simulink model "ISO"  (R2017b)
settings: Solver=FixedStepDiscrete  StartTime=0.0  StopTime=10.0  FixedStep=0.01  RelTol=1e-3  EnableMultiTasking=on
undefined symbols (not defined in the file): ASWTYPE_FALSE, ASWTYPE_TRUE, CcISO_CTCOnlineDelayTime_ms, CcISO_FirLvlDebTime_ms, CcISO_FirLvlResChrg_kohm, CcISO_FirLvlResNotChrg_kohm, CcISO_InitDiagDebMaxTi_ms, CcISO_InitDiagDebTi_ms, CcISO_IsoDefaultValue_kohm, CcISO_IsoFastDectectInsVal_kohm, CcISO_IsoFastDetectCnf_MS, CcISO_IsoFastDetectVal_kohm, CcISO_IsoMeasDelayTime_ms, CcISO_ISONegVoltDebTime_ms, CcISO_ISONegVoltFliterDiff_V, CcISO_ISOPackVoltMax_V, CcISO_ISOPackVoltMin_V, CcISO_ISOResCnfFltCnt_NUMB, CcISO_ISOResCnfFltVal_kohm, CcISO_ISOResCnfWarnCnt_NUMB, CcISO_ISOResCnfWarnVal_kohm, CcISO_ISOResNvmMin_kohm, CcISO_ISOResValueinit_kohm, CcISO_IsoResVldVal_NUMB, CcISO_ISOSlopeDelayTime_ms, CcISO_ISOSlopeFilterVal_NUMB, CcISO_NegStMeasFiltTi_ms, CcISO_NegVoltHighRat_pct, CcISO_NegVoltLowRat_pct, CcISO_NorLvlResChrg_kohm, CcISO_NorLvlResNotChrg_kohm, CcISO_PosStMeasFiltTi_ms, CcISO_ResSelfCheckDebTime_ms, CcISO_SedLvlDebTime_ms, CcISO_SedLvlResChrg_kohm, CcISO_SedLvlResNotChrg_kohm, Enum_CTCCtrCtlConnMode, Enum_CTCCtrCtlState, Enum_ISOHVIsoFltLevel, Enum_ISOHVIsoMeasState, Enum_LDPCC2St, Enum_MSMBMUState, ISO_CONST0_NUMB, ISO_CONST1000_NUMB, ISO_CONST1_NUMB, ISO_RESRB1_OHM, ISO_RESRB2_OHM, ISO_RESRS1_OHM, ISO_RESRS2_OHM, ISO_RUNTIME_MS
libraries: AIWAYS_Powertrain_BMS_lib x49
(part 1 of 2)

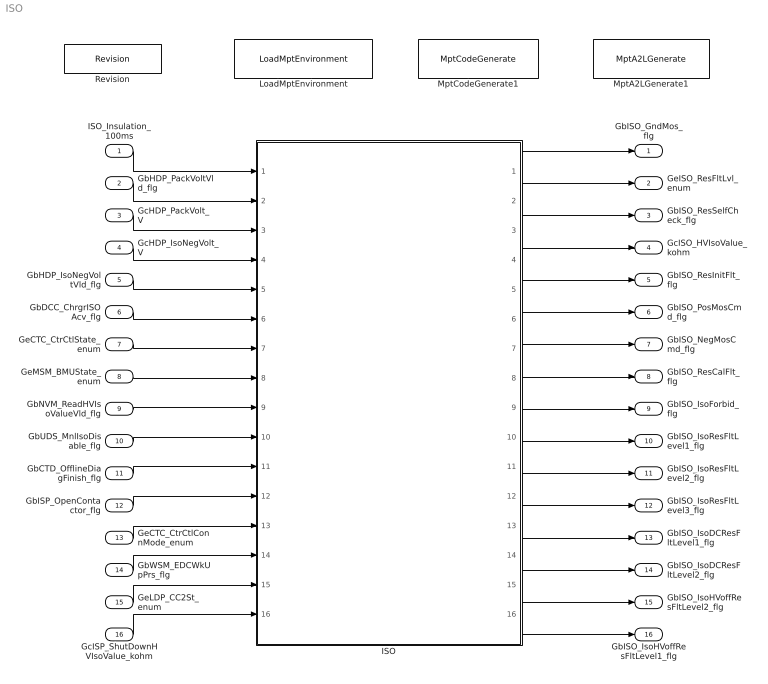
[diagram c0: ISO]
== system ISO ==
  ISO_Insulation_100ms : Inport
  GbHDP_PackVoltVld_flg : Inport  Port=2
  GcHDP_PackVolt_V : Inport  Port=3
  GcHDP_IsoNegVolt_V : Inport  Port=4
  GbHDP_IsoNegVoltVld_flg : Inport  Port=5
  GbDCC_ChrgrISOAcv_flg : Inport  Port=6
  GeCTC_CtrCtlState_enum : Inport  Port=7
  GeMSM_BMUState_enum : Inport  Port=8
  GbNVM_ReadHVIsoValueVld_flg : Inport  Port=9
  GbUDS_MnlIsoDisable_flg : Inport  Port=10
  GbCTD_OfflineDiagFinish_flg : Inport  Port=11
  GbISP_OpenContactor_flg : Inport  Port=12
  GeCTC_CtrCtlConnMode_enum : Inport  Port=13
  GbWSM_EDCWkUpPrs_flg : Inport  Port=14
  GeLDP_CC2St_enum : Inport  Port=15
  GcISP_ShutDownHVIsoValue_kohm : Inport  Port=16
  ISO : Subsystem
  LoadMptEnvironment : AIWAYS_Powertrain_BMS_lib/Config/LoadMptEnvironment  ProjectName=Comm  SuppierID=NewPlatformUAES
  MptA2LGenerate1 : AIWAYS_Powertrain_BMS_lib/Config/MptA2LGenerate  SystemSampleTime=-1
  MptCodeGenerate1 : AIWAYS_Powertrain_BMS_lib/Config/MptCodeGenerate  SystemSampleTime=-1
  Revision : AIWAYS_Powertrain_BMS_lib/Config/Revision  curVersion='M114C112R114'  newVersion='M114C112R114'
  GbISO_GndMos_flg : Outport
  GeISO_ResFltLvl_enum : Outport  Port=2
  GbISO_ResSelfCheck_flg : Outport  Port=3
  GcISO_HVIsoValue_kohm : Outport  Port=4
  GbISO_ResInitFlt_flg : Outport  Port=5
  GbISO_PosMosCmd_flg : Outport  Port=6
  GbISO_NegMosCmd_flg : Outport  Port=7
  GbISO_ResCalFlt_flg : Outport  Port=8
  GbISO_IsoForbid_flg : Outport  Port=9
  GbISO_IsoResFltLevel1_flg : Outport  Port=10
  GbISO_IsoResFltLevel2_flg : Outport  Port=11
  GbISO_IsoResFltLevel3_flg : Outport  Port=12
  GbISO_IsoDCResFltLevel1_flg : Outport  Port=13
  GbISO_IsoDCResFltLevel2_flg : Outport  Port=14
  GbISO_IsoHVoffResFltLevel2_flg : Outport  Port=15
  GbISO_IsoHVoffResFltLevel1_flg : Outport  Port=16
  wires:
  ISO_Insulation_100ms/1 -> ISO/1(ISO_Insulation_100ms)
  GbHDP_PackVoltVld_flg/1 -> ISO/2(GbHDP_PackVoltVld_flg)
  GcHDP_PackVolt_V/1 -> ISO/3(GcHDP_PackVolt_V)
  GcHDP_IsoNegVolt_V/1 -> ISO/4(GcHDP_IsoNegVolt_V)
  GbHDP_IsoNegVoltVld_flg/1 -> ISO/5(GbHDP_IsoNegVoltVld_flg)
  GbDCC_ChrgrISOAcv_flg/1 -> ISO/6(GbDCC_ChrgrISOAcv_flg)
  GeCTC_CtrCtlState_enum/1 -> ISO/7(GeCTC_CtrCtlState_enum)
  GeMSM_BMUState_enum/1 -> ISO/8(GeMSM_BMUState_enum)
  GbNVM_ReadHVIsoValueVld_flg/1 -> ISO/9(GbNVM_ReadHVIsoValueVld_flg)
  GbUDS_MnlIsoDisable_flg/1 -> ISO/10(GbUDS_MnlIsoDisable_flg)
  GbCTD_OfflineDiagFinish_flg/1 -> ISO/11(GbCTD_OfflineDiagFinish_flg)
  GbISP_OpenContactor_flg/1 -> ISO/12(GbISP_OpenContactor_flg)
  GeCTC_CtrCtlConnMode_enum/1 -> ISO/13(GeCTC_CtrCtlConnMode_enum)
  ISO/1(GbISO_GndMos_flg) -> GbISO_GndMos_flg/1
  ISO/2(GeISO_ResFltLvl_enum) -> GeISO_ResFltLvl_enum/1
  ISO/3(GbISO_ResSelfCheck_flg) -> GbISO_ResSelfCheck_flg/1
  ISO/4(GcISO_HVIsoValue_kohm) -> GcISO_HVIsoValue_kohm/1
  ISO/5(GbISO_ResInitFlt_flg) -> GbISO_ResInitFlt_flg/1
  ISO/6(GbISO_PosMosCmd_flg) -> GbISO_PosMosCmd_flg/1
  ISO/7(GbISO_NegMosCmd_flg) -> GbISO_NegMosCmd_flg/1
  ISO/8(GbISO_ResCalFlt_flg) -> GbISO_ResCalFlt_flg/1
  GbWSM_EDCWkUpPrs_flg/1 -> ISO/14(GbWSM_EDCWkUpPrs_flg)
  ISO/9(GbISO_IsoForbid_flg) -> GbISO_IsoForbid_flg/1
  ISO/10(GbISO_IsoResFltLevel1_flg) -> GbISO_IsoResFltLevel1_flg/1
  ISO/11(GbISO_IsoResFltLevel2_flg) -> GbISO_IsoResFltLevel2_flg/1
  ISO/12(GbISO_IsoResFltLevel3_flg) -> GbISO_IsoResFltLevel3_flg/1
  GeLDP_CC2St_enum/1 -> ISO/15(GeLDP_CC2St_enum)
  ISO/13(GbISO_IsoDCResFltLevel1_flg) -> GbISO_IsoDCResFltLevel1_flg/1
  ISO/14(GbISO_IsoDCResFltLevel2_flg) -> GbISO_IsoDCResFltLevel2_flg/1
  ISO/15(GbISO_IsoHVoffResFltLevel2_flg) -> GbISO_IsoHVoffResFltLevel2_flg/1
  ISO/16(GbISO_IsoHVoffResFltLevel1_flg) -> GbISO_IsoHVoffResFltLevel1_flg/1
  GcISP_ShutDownHVIsoValue_kohm/1 -> ISO/16(GcISP_ShutDownHVIsoValue_kohm)

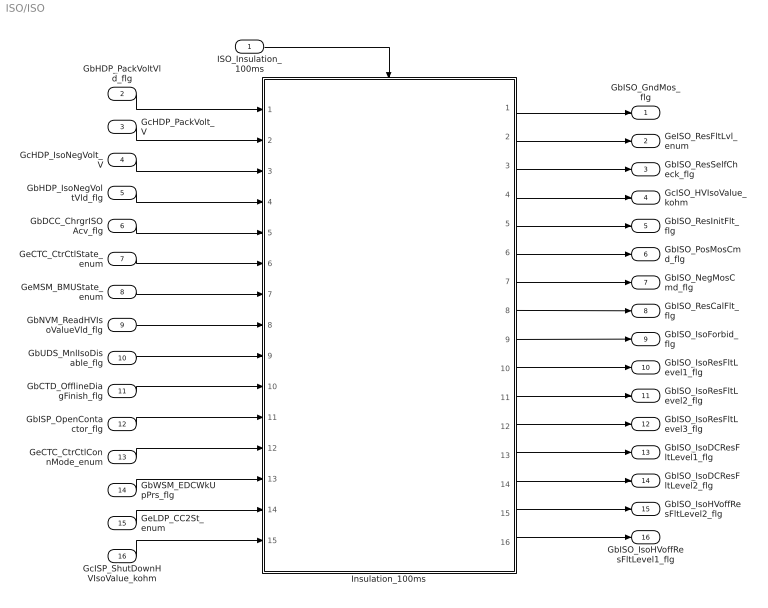
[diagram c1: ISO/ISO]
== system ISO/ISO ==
  ISO_Insulation_100ms : Inport
  GbHDP_PackVoltVld_flg : Inport  Port=2
  GcHDP_PackVolt_V : Inport  Port=3
  GcHDP_IsoNegVolt_V : Inport  Port=4
  GbHDP_IsoNegVoltVld_flg : Inport  Port=5
  GbDCC_ChrgrISOAcv_flg : Inport  Port=6
  GeCTC_CtrCtlState_enum : Inport  Port=7
  GeMSM_BMUState_enum : Inport  Port=8
  GbNVM_ReadHVIsoValueVld_flg : Inport  Port=9
  GbUDS_MnlIsoDisable_flg : Inport  Port=10
  GbCTD_OfflineDiagFinish_flg : Inport  Port=11
  GbISP_OpenContactor_flg : Inport  Port=12
  GeCTC_CtrCtlConnMode_enum : Inport  Port=13
  GbWSM_EDCWkUpPrs_flg : Inport  Port=14
  GeLDP_CC2St_enum : Inport  Port=15
  GcISP_ShutDownHVIsoValue_kohm : Inport  Port=16
  Insulation_100ms : Subsystem
  GbISO_GndMos_flg : Outport
  GeISO_ResFltLvl_enum : Outport  Port=2
  GbISO_ResSelfCheck_flg : Outport  Port=3
  GcISO_HVIsoValue_kohm : Outport  Port=4
  GbISO_ResInitFlt_flg : Outport  Port=5
  GbISO_PosMosCmd_flg : Outport  Port=6
  GbISO_NegMosCmd_flg : Outport  Port=7
  GbISO_ResCalFlt_flg : Outport  Port=8
  GbISO_IsoForbid_flg : Outport  Port=9
  GbISO_IsoResFltLevel1_flg : Outport  Port=10
  GbISO_IsoResFltLevel2_flg : Outport  Port=11
  GbISO_IsoResFltLevel3_flg : Outport  Port=12
  GbISO_IsoDCResFltLevel1_flg : Outport  Port=13
  GbISO_IsoDCResFltLevel2_flg : Outport  Port=14
  GbISO_IsoHVoffResFltLevel2_flg : Outport  Port=15
  GbISO_IsoHVoffResFltLevel1_flg : Outport  Port=16
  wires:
  ISO_Insulation_100ms/1 -> Insulation_100ms/Trigger
  Insulation_100ms/1(GbISO_GndMos_flg) -> GbISO_GndMos_flg/1
  Insulation_100ms/2(GeISO_ResFltLvl_enum) -> GeISO_ResFltLvl_enum/1
  Insulation_100ms/3(GbISO_ResSelfCheck_flg) -> GbISO_ResSelfCheck_flg/1
  Insulation_100ms/4(GcISO_HVIsoValue_kohm) -> GcISO_HVIsoValue_kohm/1
  Insulation_100ms/5(GbISO_ResInitFlt_flg) -> GbISO_ResInitFlt_flg/1
  Insulation_100ms/6(GbISO_PosMosCmd_flg) -> GbISO_PosMosCmd_flg/1
  Insulation_100ms/7(GbISO_NegMosCmd_flg) -> GbISO_NegMosCmd_flg/1
  Insulation_100ms/8(GbISO_ResCalFlt_flg) -> GbISO_ResCalFlt_flg/1
  GbHDP_PackVoltVld_flg/1 -> Insulation_100ms/1(GbHDP_PackVoltVld_flg)
  GcHDP_PackVolt_V/1 -> Insulation_100ms/2(GcHDP_PackVolt_V)
  GcHDP_IsoNegVolt_V/1 -> Insulation_100ms/3(GcHDP_IsoNegVolt_V)
  GbHDP_IsoNegVoltVld_flg/1 -> Insulation_100ms/4(GbHDP_IsoNegVoltVld_flg)
  GbDCC_ChrgrISOAcv_flg/1 -> Insulation_100ms/5(GbDCC_ChrgrISOAcv_flg)
  GeCTC_CtrCtlState_enum/1 -> Insulation_100ms/6(GeCTC_CtrCtlState_enum)
  GeMSM_BMUState_enum/1 -> Insulation_100ms/7(GeMSM_BMUState_enum)
  GbNVM_ReadHVIsoValueVld_flg/1 -> Insulation_100ms/8(GbNVM_ReadHVIsoValueVld_flg)
  GbUDS_MnlIsoDisable_flg/1 -> Insulation_100ms/9(GbUDS_MnlIsoDisable_flg)
  GbCTD_OfflineDiagFinish_flg/1 -> Insulation_100ms/10(GbCTD_OfflineDiagFinish_flg)
  GbISP_OpenContactor_flg/1 -> Insulation_100ms/11(GbISP_OpenContactor_flg)
  GeCTC_CtrCtlConnMode_enum/1 -> Insulation_100ms/12(GeCTC_CtrCtlConnMode_enum)
  GbWSM_EDCWkUpPrs_flg/1 -> Insulation_100ms/13(GbWSM_EDCWkUpPrs_flg)
  Insulation_100ms/9(GbISO_IsoForbid_flg) -> GbISO_IsoForbid_flg/1
  Insulation_100ms/10(GbISO_IsoResFltLevel1_flg) -> GbISO_IsoResFltLevel1_flg/1
  Insulation_100ms/11(GbISO_IsoResFltLevel2_flg) -> GbISO_IsoResFltLevel2_flg/1
  Insulation_100ms/12(GbISO_IsoResFltLevel3_flg) -> GbISO_IsoResFltLevel3_flg/1
  GeLDP_CC2St_enum/1 -> Insulation_100ms/14(GeLDP_CC2St_enum)
  Insulation_100ms/13(GbISO_IsoDCResFltLevel1_flg) -> GbISO_IsoDCResFltLevel1_flg/1
  Insulation_100ms/14(GbISO_IsoDCResFltLevel2_flg) -> GbISO_IsoDCResFltLevel2_flg/1
  Insulation_100ms/15(GbISO_IsoHVoffResFltLevel2_flg) -> GbISO_IsoHVoffResFltLevel2_flg/1
  Insulation_100ms/16(GbISO_IsoHVoffResFltLevel1_flg) -> GbISO_IsoHVoffResFltLevel1_flg/1
  GcISP_ShutDownHVIsoValue_kohm/1 -> Insulation_100ms/15(GcISP_ShutDownHVIsoValue_kohm)

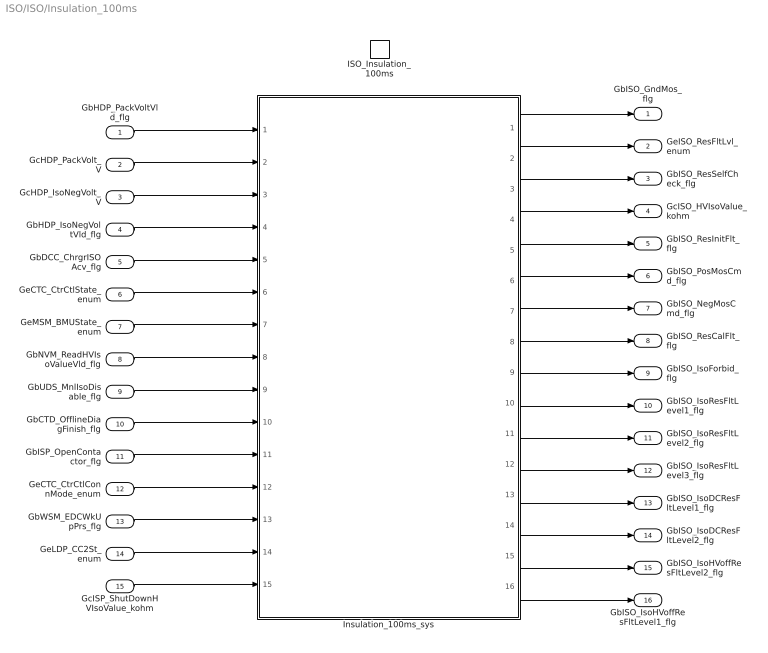
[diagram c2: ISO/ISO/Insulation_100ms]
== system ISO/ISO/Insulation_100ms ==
  GbHDP_PackVoltVld_flg : Inport
  GcHDP_PackVolt_V : Inport  Port=2
  GcHDP_IsoNegVolt_V : Inport  Port=3
  GbHDP_IsoNegVoltVld_flg : Inport  Port=4
  GbDCC_ChrgrISOAcv_flg : Inport  Port=5
  GeCTC_CtrCtlState_enum : Inport  Port=6
  GeMSM_BMUState_enum : Inport  Port=7
  GbNVM_ReadHVIsoValueVld_flg : Inport  Port=8
  GbUDS_MnlIsoDisable_flg : Inport  Port=9
  GbCTD_OfflineDiagFinish_flg : Inport  Port=10
  GbISP_OpenContactor_flg : Inport  Port=11
  GeCTC_CtrCtlConnMode_enum : Inport  Port=12
  GbWSM_EDCWkUpPrs_flg : Inport  Port=13
  GeLDP_CC2St_enum : Inport  Port=14
  GcISP_ShutDownHVIsoValue_kohm : Inport  Port=15
  ISO_Insulation_100ms : TriggerPort  TriggerType=function-call  VariantControl=(inherit)
  Insulation_100ms_sys : Subsystem
  GbISO_GndMos_flg : Outport
  GeISO_ResFltLvl_enum : Outport  Port=2
  GbISO_ResSelfCheck_flg : Outport  Port=3
  GcISO_HVIsoValue_kohm : Outport  Port=4
  GbISO_ResInitFlt_flg : Outport  Port=5
  GbISO_PosMosCmd_flg : Outport  Port=6
  GbISO_NegMosCmd_flg : Outport  Port=7
  GbISO_ResCalFlt_flg : Outport  Port=8
  GbISO_IsoForbid_flg : Outport  Port=9
  GbISO_IsoResFltLevel1_flg : Outport  Port=10
  GbISO_IsoResFltLevel2_flg : Outport  Port=11
  GbISO_IsoResFltLevel3_flg : Outport  Port=12
  GbISO_IsoDCResFltLevel1_flg : Outport  Port=13
  GbISO_IsoDCResFltLevel2_flg : Outport  Port=14
  GbISO_IsoHVoffResFltLevel2_flg : Outport  Port=15
  GbISO_IsoHVoffResFltLevel1_flg : Outport  Port=16
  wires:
  Insulation_100ms_sys/1(GbISO_GndMos_flg) -> GbISO_GndMos_flg/1
  Insulation_100ms_sys/2(GeISO_ResFltLvl_enum) -> GeISO_ResFltLvl_enum/1
  Insulation_100ms_sys/3(GbISO_ResSelfCheck_flg) -> GbISO_ResSelfCheck_flg/1
  Insulation_100ms_sys/4(GcISO_HVIsoValue_kohm) -> GcISO_HVIsoValue_kohm/1
  Insulation_100ms_sys/5(GbISO_ResInitFlt_flg) -> GbISO_ResInitFlt_flg/1
  Insulation_100ms_sys/6(GbISO_PosMosCmd_flg) -> GbISO_PosMosCmd_flg/1
  Insulation_100ms_sys/7(GbISO_NegMosCmd_flg) -> GbISO_NegMosCmd_flg/1
  Insulation_100ms_sys/8(GbISO_ResCalFlt_flg) -> GbISO_ResCalFlt_flg/1
  GbHDP_PackVoltVld_flg/1 -> Insulation_100ms_sys/1(GbHDP_PackVoltVld_flg)
  GcHDP_PackVolt_V/1 -> Insulation_100ms_sys/2(GcHDP_PackVolt_V)
  GcHDP_IsoNegVolt_V/1 -> Insulation_100ms_sys/3(GcHDP_IsoNegVolt_V)
  GbHDP_IsoNegVoltVld_flg/1 -> Insulation_100ms_sys/4(GbHDP_IsoNegVoltVld_flg)
  GbDCC_ChrgrISOAcv_flg/1 -> Insulation_100ms_sys/5(GbDCC_ChrgrISOAcv_flg)
  GeCTC_CtrCtlState_enum/1 -> Insulation_100ms_sys/6(GeCTC_CtrCtlState_enum)
  GeMSM_BMUState_enum/1 -> Insulation_100ms_sys/7(GeMSM_BMUState_enum)
  GbNVM_ReadHVIsoValueVld_flg/1 -> Insulation_100ms_sys/8(GbNVM_ReadHVIsoValueVld_flg)
  GbUDS_MnlIsoDisable_flg/1 -> Insulation_100ms_sys/9(GbUDS_MnlIsoDisable_flg)
  GbCTD_OfflineDiagFinish_flg/1 -> Insulation_100ms_sys/10(GbCTD_OfflineDiagFinish_flg)
  GbISP_OpenContactor_flg/1 -> Insulation_100ms_sys/11(GbISP_OpenContactor_flg)
  GeCTC_CtrCtlConnMode_enum/1 -> Insulation_100ms_sys/12(GeCTC_CtrCtlConnMode_enum)
  GbWSM_EDCWkUpPrs_flg/1 -> Insulation_100ms_sys/13(GbWSM_EDCWkUpPrs_flg)
  Insulation_100ms_sys/9(GbISO_IsoForbid_flg) -> GbISO_IsoForbid_flg/1
  Insulation_100ms_sys/10(GbISO_IsoResFltLevel1_flg) -> GbISO_IsoResFltLevel1_flg/1
  Insulation_100ms_sys/11(GbISO_IsoResFltLevel2_flg) -> GbISO_IsoResFltLevel2_flg/1
  Insulation_100ms_sys/12(GbISO_IsoResFltLevel3_flg) -> GbISO_IsoResFltLevel3_flg/1
  GeLDP_CC2St_enum/1 -> Insulation_100ms_sys/14(GeLDP_CC2St_enum)
  Insulation_100ms_sys/13(GbISO_IsoDCResFltLevel1_flg) -> GbISO_IsoDCResFltLevel1_flg/1
  Insulation_100ms_sys/14(GbISO_IsoDCResFltLevel2_flg) -> GbISO_IsoDCResFltLevel2_flg/1
  Insulation_100ms_sys/15(GbISO_IsoHVoffResFltLevel2_flg) -> GbISO_IsoHVoffResFltLevel2_flg/1
  Insulation_100ms_sys/16(GbISO_IsoHVoffResFltLevel1_flg) -> GbISO_IsoHVoffResFltLevel1_flg/1
  GcISP_ShutDownHVIsoValue_kohm/1 -> Insulation_100ms_sys/15(GcISP_ShutDownHVIsoValue_kohm)

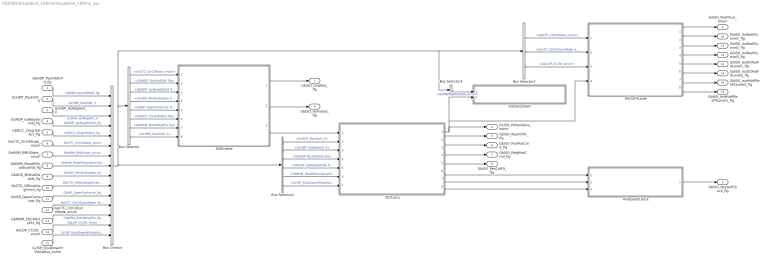
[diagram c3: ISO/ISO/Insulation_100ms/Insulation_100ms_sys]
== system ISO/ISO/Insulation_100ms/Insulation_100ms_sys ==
  GbHDP_PackVoltVld_flg : Inport
  GcHDP_PackVolt_V : Inport  Port=2
  GcHDP_IsoNegVolt_V : Inport  Port=3
  GbHDP_IsoNegVoltVld_flg : Inport  Port=4
  GbDCC_ChrgrISOAcv_flg : Inport  Port=5
  GeCTC_CtrCtlState_enum : Inport  Port=6
  GeMSM_BMUState_enum : Inport  Port=7
  GbNVM_ReadHVIsoValueVld_flg : Inport  Port=8
  GbUDS_MnlIsoDisable_flg : Inport  Port=9
  GbCTD_OfflineDiagFinish_flg : Inport  Port=10
  GbISP_OpenContactor_flg : Inport  Port=11
  GeCTC_CtrCtlConnMode_enum : Inport  Port=12
  GbWSM_EDCWkUpPrs_flg : Inport  Port=13
  GeLDP_CC2St_enum : Inport  Port=14
  GcISP_ShutDownHVIsoValue_kohm : Inport  Port=15
  Bus Creator : BusCreator  Inputs=15
  Bus Selector : BusSelector  OutputSignals=GeCTC_CtrCtlState_enum,GbHDP_PackVoltVld_flg,GbHDP_IsoNegVoltVld_flg,GbUDS_MnlIsoDisable_flg,GbISP_OpenContactor_flg,GbDCC_ChrgrISOAcv_flg,GbWSM_EDCWkUpPrs_flg,GcHDP_PackVolt_V
  Bus Selector1 : BusSelector  OutputSignals=GcHDP_PackVolt_V,GcHDP_IsoNegVolt_V,GbHDP_PackVoltVld_flg,GbHDP_IsoNegVoltVld_flg,GbNVM_ReadHVIsoValueVld_flg,GcISP_ShutDownHVIsoValue_kohm
  Bus Selector2 : BusSelector  OutputSignals=GeCTC_CtrCtlState_enum,GeCTC_CtrCtlConnMode_enum,GeLDP_CC2St_enum
  Bus Selector3 : BusSelector  OutputSignals=GeMSM_BMUState_enum
  DataStoreISO : Subsystem
  HVIsoFltLevel : Subsystem
  HVIsoSelfCheck : Subsystem
  ISOCalcu : Subsystem
  ISOEnable : Subsystem
  GbISO_GndMos_flg : Outport
  GeISO_ResFltLvl_enum : Outport  Port=2
  GbISO_ResSelfCheck_flg : Outport  Port=3
  GcISO_HVIsoValue_kohm : Outport  Port=4
  GbISO_ResInitFlt_flg : Outport  Port=5
  GbISO_PosMosCmd_flg : Outport  Port=6
  GbISO_NegMosCmd_flg : Outport  Port=7
  GbISO_ResCalFlt_flg : Outport  Port=8
  GbISO_IsoForbid_flg : Outport  Port=9
  GbISO_IsoResFltLevel1_flg : Outport  Port=10
  GbISO_IsoResFltLevel2_flg : Outport  Port=11
  GbISO_IsoResFltLevel3_flg : Outport  Port=12
  GbISO_IsoDCResFltLevel1_flg : Outport  Port=13
  GbISO_IsoDCResFltLevel2_flg : Outport  Port=14
  GbISO_IsoHVoffResFltLevel2_flg : Outport  Port=15
  GbISO_IsoHVoffResFltLevel1_flg : Outport  Port=16
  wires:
  GbHDP_PackVoltVld_flg/1 -> Bus Creator/1  "GbHDP_PackVoltVld_flg"
  GcHDP_PackVolt_V/1 -> Bus Creator/2  "GcHDP_PackVolt_V"
  GcHDP_IsoNegVolt_V/1 -> Bus Creator/3  "GcHDP_IsoNegVolt_V"
  GbHDP_IsoNegVoltVld_flg/1 -> Bus Creator/4  "GbHDP_IsoNegVoltVld_flg"
  GbDCC_ChrgrISOAcv_flg/1 -> Bus Creator/5  "GbDCC_ChrgrISOAcv_flg"
  GeCTC_CtrCtlState_enum/1 -> Bus Creator/6  "GeCTC_CtrCtlState_enum"
  GeMSM_BMUState_enum/1 -> Bus Creator/7  "GeMSM_BMUState_enum"
  GbNVM_ReadHVIsoValueVld_flg/1 -> Bus Creator/8  "GbNVM_ReadHVIsoValueVld_flg"
  GbUDS_MnlIsoDisable_flg/1 -> Bus Creator/9  "GbUDS_MnlIsoDisable_flg"
  GbCTD_OfflineDiagFinish_flg/1 -> Bus Creator/10  "GbCTD_OfflineDiagFinish_flg"
  Bus Selector/1 -> ISOEnable/1(GeCTC_CtrCtlState_enum)  "<GeCTC_CtrCtlState_enum>"
  Bus Selector/2 -> ISOEnable/2(GbHDP_PackVoltVld_flg)  "<GbHDP_PackVoltVld_flg>"
  Bus Selector/3 -> ISOEnable/3(GbHDP_IsoNegVoltVld_flg)  "<GbHDP_IsoNegVoltVld_flg>"
  Bus Selector/4 -> ISOEnable/4(GbUDS_MnlIsoDisable_flg)  "<GbUDS_MnlIsoDisable_flg>"
  Bus Selector/5 -> ISOEnable/5(GbISP_OpenContactor_flg)  "<GbISP_OpenContactor_flg>"
  Bus Selector/6 -> ISOEnable/6(GbDCC_ChrgrISOAcv_flg)  "<GbDCC_ChrgrISOAcv_flg>"
  ISOEnable/3(LbISO_IsoForbid_flg) -> ISOCalcu/1(LbISO_IsoForbid_flg)
  Bus Selector1/1 -> ISOCalcu/2(GcHDP_PackVolt_V)  "<GcHDP_PackVolt_V>"
  Bus Selector1/2 -> ISOCalcu/3(GcHDP_IsoNegVolt_V)  "<GcHDP_IsoNegVolt_V>"
  Bus Selector1/3 -> ISOCalcu/4(GbHDP_PackVoltVld_flg)  "<GbHDP_PackVoltVld_flg>"
  Bus Selector1/4 -> ISOCalcu/5(GbHDP_IsoNegVoltVld_flg)  "<GbHDP_IsoNegVoltVld_flg>"
  ISOEnable/1(GbISO_GndMos_flg) -> GbISO_GndMos_flg/1
  Bus Selector1/5 -> ISOCalcu/6(GbNVM_ReadHVIsoValueVld_flg)  "<GbNVM_ReadHVIsoValueVld_flg>"
  ISOCalcu/1(GcISO_HVIsoValue_kohm) -> DataStoreISO/2(GcISO_HVIsoValue_kohm), HVIsoFltLevel/4(GcISO_HVIsoValue_kohm), GcISO_HVIsoValue_kohm/1
  GeCTC_CtrCtlConnMode_enum/1 -> Bus Creator/12  "GeCTC_CtrCtlConnMode_enum"
  Bus Selector2/1 -> HVIsoFltLevel/1(GeCTC_CtrCtlState_enum)  "<GeCTC_CtrCtlState_enum>"
  Bus Selector2/2 -> HVIsoFltLevel/2(GeCTC_CtrCtlConnMode_enum)  "<GeCTC_CtrCtlConnMode_enum>"
  Bus Creator/1 -> Bus Selector3/1, Bus Selector2/1, Bus Selector/1, Bus Selector1/1
  Bus Selector3/1 -> DataStoreISO/1(GeMSM_BMUState_enum)  "<GeMSM_BMUState_enum>"
  HVIsoFltLevel/1(GeISO_ResFltLvl_enum) -> GeISO_ResFltLvl_enum/1
  HVIsoSelfCheck/1(GbISO_ResSelfCheck_flg) -> GbISO_ResSelfCheck_flg/1
  ISOCalcu/2(GbISO_ResInitFlt_flg) -> GbISO_ResInitFlt_flg/1
  ISOCalcu/3(GbISO_PosMosCmd_flg) -> GbISO_PosMosCmd_flg/1
  ISOCalcu/4(GbISO_NegMosCmd_flg) -> GbISO_NegMosCmd_flg/1
  ISOCalcu/5(GbISO_ResCalFlt_flg) -> GbISO_ResCalFlt_flg/1
  GbWSM_EDCWkUpPrs_flg/1 -> Bus Creator/13  "GbWSM_EDCWkUpPrs_flg"
  Bus Selector/7 -> ISOEnable/7(GbWSM_EDCWkUpPrs_flg)  "<GbWSM_EDCWkUpPrs_flg>"
  ISOEnable/2(GbISO_IsoForbid_flg) -> GbISO_IsoForbid_flg/1
  HVIsoFltLevel/2(GbISO_IsoResFltLevel1_flg) -> GbISO_IsoResFltLevel1_flg/1
  HVIsoFltLevel/3(GbISO_IsoResFltLevel2_flg) -> GbISO_IsoResFltLevel2_flg/1
  HVIsoFltLevel/4(GbISO_IsoResFltLevel3_flg) -> GbISO_IsoResFltLevel3_flg/1
  Bus Selector/8 -> ISOEnable/8(" GcHDP_PackVolt_V")  "<GcHDP_PackVolt_V>"
  GbISP_OpenContactor_flg/1 -> Bus Creator/11  "GbISP_OpenContactor_flg"
  GeLDP_CC2St_enum/1 -> Bus Creator/14  "GeLDP_CC2St_enum"
  Bus Selector2/3 -> HVIsoFltLevel/3(GeLDP_CC2St_enum)  "<GeLDP_CC2St_enum>"
  HVIsoFltLevel/5(GbISO_IsoDCResFltLevel1_flg) -> GbISO_IsoDCResFltLevel1_flg/1
  HVIsoFltLevel/6(GbISO_IsoDCResFltLevel2_flg) -> GbISO_IsoDCResFltLevel2_flg/1
  HVIsoFltLevel/7(GbISO_IsoHVoffResFltLevel2_flg) -> GbISO_IsoHVoffResFltLevel2_flg/1
  HVIsoFltLevel/8(GbISO_IsoHVoffResFltLevel1_flg) -> GbISO_IsoHVoffResFltLevel1_flg/1
  ISOCalcu/6(LbISO_InitNegVoltCheck_flg) -> HVIsoSelfCheck/1(LbISO_InitNegVoltCheck_flg)
  ISOCalcu/7(LbISO_IsoFastDetectEna_flg) -> HVIsoSelfCheck/2(LbISO_IsoFastDetectEna_flg)
  GcISP_ShutDownHVIsoValue_kohm/1 -> Bus Creator/15  "GcISP_ShutDownHVIsoValue_kohm"
  Bus Selector1/6 -> ISOCalcu/7(GcISP_ShutDownHVIsoValue_kohm)  "<GcISP_ShutDownHVIsoValue_kohm>"
  ISOCalcu/8(LcISO_HVIsoValue_kohm) -> HVIsoSelfCheck/3(LcISO_HVIsoValue_kohm)

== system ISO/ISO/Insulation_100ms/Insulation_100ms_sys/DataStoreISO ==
  GeMSM_BMUState_enum : Inport
  GcISO_HVIsoValue_kohm : Inport  Port=2
  Constant3 : Constant  Value=Enum_MSMBMUState.Enum_MSMBMUState_Shutdown
  Data Type Conversion1 : DataTypeConversion
  DataStoreISO_Work : Subsystem
  Relational Operator3 : RelationalOperator  Operator===  OutDataTypeStr=boolean
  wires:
  GcISO_HVIsoValue_kohm/1 -> DataStoreISO_Work/1(GcISO_HVIsoValue_kohm)
  GeMSM_BMUState_enum/1 -> Data Type Conversion1/1
  Relational Operator3/1 -> DataStoreISO_Work/Enable  "LbISO_DataStoreEN_flg"
  Constant3/1 -> Relational Operator3/2
  Data Type Conversion1/1 -> Relational Operator3/1

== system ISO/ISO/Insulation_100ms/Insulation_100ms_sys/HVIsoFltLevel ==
  GeCTC_CtrCtlState_enum : Inport
  GeCTC_CtrCtlConnMode_enum : Inport  Port=2
  GeLDP_CC2St_enum : Inport  Port=3
  GcISO_HVIsoValue_kohm : Inport  Port=4
  ISOFlt : Subsystem
  IsoLevelResThrld : Subsystem
  GeISO_ResFltLvl_enum : Outport
  GbISO_IsoResFltLevel1_flg : Outport  Port=2
  GbISO_IsoResFltLevel2_flg : Outport  Port=3
  GbISO_IsoResFltLevel3_flg : Outport  Port=4
  GbISO_IsoDCResFltLevel1_flg : Outport  Port=5
  GbISO_IsoDCResFltLevel2_flg : Outport  Port=6
  GbISO_IsoHVoffResFltLevel2_flg : Outport  Port=7
  GbISO_IsoHVoffResFltLevel1_flg : Outport  Port=8
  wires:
  GcISO_HVIsoValue_kohm/1 -> ISOFlt/1(GcISO_HVIsoValue_kohm)
  GeCTC_CtrCtlState_enum/1 -> IsoLevelResThrld/1(GeCTC_CtrCtlState_enum), ISOFlt/3(GeCTC_CtrCtlState_enum)
  IsoLevelResThrld/1(LcISO_IsoSecondLevelResThrld_kohm) -> ISOFlt/4(LcISO_IsoSecondLevelResThrld_kohm)
  IsoLevelResThrld/2(LcISO_IsoFirstLevelResThrld_kohm) -> ISOFlt/5(LcISO_IsoFirstLevelResThrld_kohm)
  IsoLevelResThrld/3(LcISO_IsoNormalLevelResThrld_kohm) -> ISOFlt/6(LcISO_IsoNormalLevelResThrld_kohm)
  GeCTC_CtrCtlConnMode_enum/1 -> IsoLevelResThrld/2(GeCTC_CtrCtlConnMode_enum)
  ISOFlt/1(GeISO_ResFltLvl_enum) -> GeISO_ResFltLvl_enum/1
  ISOFlt/2(GbISO_IsoResFltLevel1_flg) -> GbISO_IsoResFltLevel1_flg/1
  ISOFlt/3(GbISO_IsoResFltLevel2_flg) -> GbISO_IsoResFltLevel2_flg/1
  ISOFlt/4(GbISO_IsoResFltLevel3_flg) -> GbISO_IsoResFltLevel3_flg/1
  GeLDP_CC2St_enum/1 -> ISOFlt/2(GeLDP_CC2St_enum)
  ISOFlt/5(GbISO_IsoDCResFltLevel1_flg) -> GbISO_IsoDCResFltLevel1_flg/1
  ISOFlt/6(GbISO_IsoDCResFltLevel2_flg) -> GbISO_IsoDCResFltLevel2_flg/1
  ISOFlt/7(GbISO_IsoHVoffResFltLevel2_flg) -> GbISO_IsoHVoffResFltLevel2_flg/1
  ISOFlt/8(GbISO_IsoHVoffResFltLevel1_flg) -> GbISO_IsoHVoffResFltLevel1_flg/1

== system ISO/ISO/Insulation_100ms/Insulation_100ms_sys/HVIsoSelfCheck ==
  LbISO_InitNegVoltCheck_flg : Inport
  LbISO_IsoFastDetectEna_flg : Inport  Port=2
  LcISO_HVIsoValue_kohm : Inport  Port=3
  BMSDebounceStartZero : AIWAYS_Powertrain_BMS_lib/Debounce & Delay/BMSDebounceStartZero
  Comparison : RelationalOperator  Operator=>  OutDataTypeStr=boolean
  Comparison1 : RelationalOperator  Operator===  OutDataTypeStr=boolean
  Comparison2 : RelationalOperator  Operator===  OutDataTypeStr=boolean
  Comparison4 : RelationalOperator  Operator===  OutDataTypeStr=boolean
  Constant1 : Constant  Value=ASWTYPE_TRUE
  Constant2 : Constant  Value=ASWTYPE_TRUE
  Constant3 : Constant  Value=ASWTYPE_FALSE
  Constant4 : Constant  Value=CcISO_ResSelfCheckDebTime_ms
  Constant5 : Constant  Value=ISO_RUNTIME_MS
  Constant6 : Constant  Value=ISO_RUNTIME_MS
  Constant7 : Constant  Value=CcISO_ResSelfCheckDebTime_ms
  Constant8 : Constant  Value=CcISO_ISOResCnfFltVal_kohm
  ISO_GbISO_ResSelfCheck_flg : AIWAYS_Powertrain_BMS_lib/Signals/OverWrite  OverWrite_Value=CbISO_ResSelfCheckOvr_flg  OverWrite_flag=CbISO_ResSelfCheckOvrSwt_flg
  Logical : Logic  OutDataTypeStr=boolean
  Logical1 : Logic  Operator=OR  Inputs=3  OutDataTypeStr=boolean
  GbISO_ResSelfCheck_flg : Outport
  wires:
  Logical1/1 -> BMSDebounceStartZero/1
  ISO_GbISO_ResSelfCheck_flg/1 -> GbISO_ResSelfCheck_flg/1  "GbISO_ResSelfCheck_flg"
  Constant1/1 -> Comparison4/2
  Constant2/1 -> Comparison1/2
  LbISO_InitNegVoltCheck_flg/1 -> Comparison1/1
  Comparison4/1 -> Logical/2
  Comparison1/1 -> Logical/1
  Logical/1 -> Logical1/1
  Comparison2/1 -> Logical1/2
  Constant3/1 -> Comparison2/2
  LbISO_IsoFastDetectEna_flg/1 -> Comparison4/1, Comparison2/1
  BMSDebounceStartZero/1 -> ISO_GbISO_ResSelfCheck_flg/1
  Constant6/1 -> BMSDebounceStartZero/3
  Constant4/1 -> BMSDebounceStartZero/2
  Constant5/1 -> BMSDebounceStartZero/5
  Constant7/1 -> BMSDebounceStartZero/4
  LcISO_HVIsoValue_kohm/1 -> Comparison/1
  Comparison/1 -> Logical1/3
  Constant8/1 -> Comparison/2

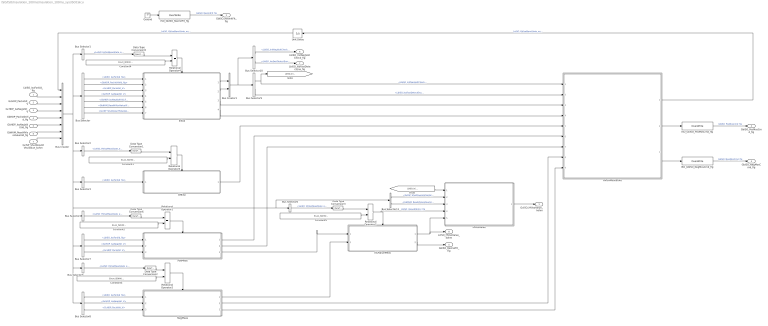
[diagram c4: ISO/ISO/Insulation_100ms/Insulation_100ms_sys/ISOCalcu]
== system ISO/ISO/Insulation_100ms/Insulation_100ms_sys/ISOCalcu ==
  LbISO_IsoForbid_flg : Inport
  GcHDP_PackVolt_V : Inport  Port=2
  GcHDP_IsoNegVolt_V : Inport  Port=3
  GbHDP_PackVoltVld_flg : Inport  Port=4
  GbHDP_IsoNegVoltVld_flg : Inport  Port=5
  GbNVM_ReadHVIsoValueVld_flg : Inport  Port=6
  GcISP_ShutDownHVIsoValue_kohm : Inport  Port=7
  Bus Creator : BusCreator  Inputs=8
  Bus Creator1 : BusCreator  Inputs=2
  Bus Selector : BusSelector  OutputSignals=LbISO_IsoForbid_flg,GbHDP_PackVoltVld_flg,GcHDP_PackVolt_V,GcHDP_IsoNegVolt_V,GbHDP_IsoNegVoltVld_flg,GbNVM_ReadHVIsoValueVld_flg,GcISP_ShutDownHVIsoValue_kohm
  Bus Selector{1..2,4..6} (5 alike) : BusSelector  OutputSignals=LeISO_HVIsoMeasState_enum
  Bus Selector10 : BusSelector  OutputSignals=LbISO_InitNegVoltCheck_flg,LbISO_IsoFastDetectEna_flg
  Bus Selector11 : BusSelector  OutputSignals=GcISP_ShutDownHVIsoValue_kohm,GbNVM_ReadHVIsoValueVld_flg
  Bus Selector3 : BusSelector  OutputSignals=LbISO_IsoForbid_flg
  Bus Selector7 : BusSelector  OutputSignals=LbISO_IsoForbid_flg,GcHDP_IsoNegVolt_V,GcHDP_PackVolt_V
  Bus Selector8 : BusSelector  OutputSignals=LbISO_IsoForbid_flg,GcHDP_IsoNegVolt_V,GcHDP_PackVolt_V
  Bus Selector9 : BusSelector  OutputSignals=LbISO_InitNegVoltCheck_flg,LbISO_IsoFastDetectEna_flg
  Constant1 : Constant  Value=Enum_ISOHVIsoMeasState.Enum_ISOHVIsoMeasState_Offline
  Constant2 : Constant  Value=Enum_ISOHVIsoMeasState.Enum_ISOHVIsoMeasState_PosMeas
  Constant3 : Constant  Value=Enum_ISOHVIsoMeasState.Enum_ISOHVIsoMeasState_NegMeas
  Constant4 : Constant  Value=Enum_ISOHVIsoMeasState.Enum_ISOHVIsoMeasState_Initial
  Constant5 : Constant  Value=Enum_ISOHVIsoMeasState.Enum_ISOHVIsoMeasState_VauleCalcu
  Data Type Conversion{1..3,5..6} (5 alike) : DataTypeConversion
  Ground : Ground
  HVIsoMeasState : Stateflow chart  TreatAsAtomicUnit=on
  HVIsoValue : Subsystem
  ISOValueMeas : Subsystem  TreatAsAtomicUnit=on
  ISO_GbISO_NegMosCmd_flg : AIWAYS_Powertrain_BMS_lib/Signals/OverWrite  OverWrite_Value=CbISO_NegMosCmdOvr_flg  OverWrite_flag=CbISO_NegMosCmdOvrSwt_flg
  ISO_GbISO_PosMosCmd_flg : AIWAYS_Powertrain_BMS_lib/Signals/OverWrite  OverWrite_Value=CbISO_PosMosCmdOvr_flg  OverWrite_flag=CbISO_PosMosCmdOvrSwt_flg
  ISO_GbISO_ResInitFlt_flg : AIWAYS_Powertrain_BMS_lib/Signals/OverWrite  OverWrite_Value=CbISO_ResInitFltOvr_flg  OverWrite_flag=CbISO_ResInitFltOvrSwt_flg
  Initial : Subsystem  TreatAsAtomicUnit=on
  NegMeas : Subsystem  TreatAsAtomicUnit=on
  Offline : Subsystem  TreatAsAtomicUnit=on
  PosMeas : Subsystem  TreatAsAtomicUnit=on
  Relational Operator{1..5} (5 alike) : RelationalOperator  Operator===  OutDataTypeStr=boolean
  Unit Delay : UnitDelay  SampleTime=-1  StateName=StateName
  GcISO_HVIsoValue_kohm : Outport
  GbISO_ResInitFlt_flg : Outport  Port=2
  GbISO_PosMosCmd_flg : Outport  Port=3
  GbISO_NegMosCmd_flg : Outport  Port=4
  GbISO_ResCalFlt_flg : Outport  Port=5
  LbISO_InitNegVoltCheck_flg : Outport  Port=6
  LbISO_IsoFastDetectEna_flg : Outport  Port=7
  LcISO_HVIsoValue_kohm : Outport  Port=8
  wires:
  Relational Operator1/1 -> PosMeas/Enable
  Relational Operator2/1 -> NegMeas/Enable
  Constant2/1 -> Relational Operator1/2
  Constant3/1 -> Relational Operator2/2
  HVIsoMeasState/2(GbISO_PosMosCmd_flg) -> ISO_GbISO_PosMosCmd_flg/1
  HVIsoMeasState/3(GbISO_NegMosCmd_flg) -> ISO_GbISO_NegMosCmd_flg/1
  ISOValueMeas/1(LcISO_HVIsoValue_kohm) -> LcISO_HVIsoValue_kohm/1, HVIsoValue/5(LcISO_HVIsoValue_kohm)
  HVIsoMeasState/1(LeISO_HVIsoMeasState_enum) -> Unit Delay/1  "LeISO_HVIsoMeasState_enum"
  Data Type Conversion6/1 -> Relational Operator1/1
  Data Type Conversion2/1 -> Relational Operator2/1
  PosMeas/3(LcISO_PosStBeta_numb) -> ISOValueMeas/1(LcISO_PosStBeta_numb)
  NegMeas/1(LcISO_NegStAlpha_numb) -> ISOValueMeas/2(LcISO_NegStAlpha_numb)
  HVIsoValue/1(GcISO_HVIsoValue_kohm) -> GcISO_HVIsoValue_kohm/1
  LbISO_IsoForbid_flg/1 -> Bus Creator/2
  GcHDP_PackVolt_V/1 -> Bus Creator/3
  GcHDP_IsoNegVolt_V/1 -> Bus Creator/4
  GbHDP_PackVoltVld_flg/1 -> Bus Creator/5
  GbHDP_IsoNegVoltVld_flg/1 -> Bus Creator/6
  Unit Delay/1 -> Bus Creator/1  "LeISO_HVIsoMeasState_enum"
  Bus Selector/1 -> Initial/1(LbISO_IsoForbid_flg)  "<LbISO_IsoForbid_flg>"
  Bus Selector/2 -> Initial/2(GbHDP_PackVoltVld_flg)  "<GbHDP_PackVoltVld_flg>"
  Bus Selector/3 -> Initial/3(GcHDP_PackVolt_V)  "<GcHDP_PackVolt_V>"
  Bus Selector/4 -> Initial/4(GcHDP_IsoNegVolt_V)  "<GcHDP_IsoNegVolt_V>"
  Bus Selector/5 -> Initial/5(GbHDP_IsoNegVoltVld_flg)  "<GbHDP_IsoNegVoltVld_flg>"
  Relational Operator4/1 -> Initial/Enable
  Constant4/1 -> Relational Operator4/2
  Data Type Conversion5/1 -> Relational Operator4/1
  Bus Selector1/1 -> Data Type Conversion5/1  "<LeISO_HVIsoMeasState_enum>"
  Bus Selector2/1 -> Data Type Conversion1/1  "<LeISO_HVIsoMeasState_enum>"
  Data Type Conversion1/1 -> Relational Operator5/1
  Constant1/1 -> Relational Operator5/2
  Relational Operator5/1 -> Offline/Enable
  Bus Selector3/1 -> Offline/1(LbISO_IsoForbid_flg)  "<LbISO_IsoForbid_flg>"
  Bus Selector4/1 -> Data Type Conversion6/1  "<LeISO_HVIsoMeasState_enum>"
  Bus Selector5/1 -> Data Type Conversion2/1  "<LeISO_HVIsoMeasState_enum>"
  Bus Selector6/1 -> Data Type Conversion3/1  "<LeISO_HVIsoMeasState_enum>"
  Bus Creator/1 -> Bus Selector1/1, Bus Selector/1, Bus Selector8/1, Bus Selector5/1, Bus Selector7/1, Bus Selector4/1, Bus Selector11/1, Bus Selector6/1, Bus Selector3/1, Bus Selector2/1
  Data Type Conversion3/1 -> Relational Operator3/1
  Constant5/1 -> Relational Operator3/2
  Relational Operator3/1 -> HVIsoValue/4(LbISO_ValueStEntry_flg), ISOValueMeas/Enable  "LbISO_ValueStEntry_flg"
  Initial/3(LbISO_InitiaStMosCmd_flg) -> HVIsoMeasState/3(LbISO_InitiaStMosCmd_flg)
  Initial/4(LbISO_Init2Offline_flg) -> HVIsoMeasState/4(LbISO_Init2Offline_flg)
  Offline/1(LbISO_Offline2PosMeas_flg) -> HVIsoMeasState/5(LbISO_Offline2PosMeas_flg)
  PosMeas/1(LbISO_PosMeas2NegMeas_flg) -> HVIsoMeasState/6(LbISO_PosMeas2NegMeas_flg)
  PosMeas/2(LbISO_PosMeas2Offline_flg) -> HVIsoMeasState/7(LbISO_PosMeas2Offline_flg)
  NegMeas/2(LbISO_NegMeas2VauleCalcu_flg) -> HVIsoMeasState/8(LbISO_NegMeas2VauleCalcu_flg)
  NegMeas/3(LbISO_NegMeas2Offline_flg) -> HVIsoMeasState/9(LbISO_NegMeas2Offline_flg)
  Bus Selector7/1 -> PosMeas/1(LbISO_IsoForbid_flg)  "<LbISO_IsoForbid_flg>"
  Bus Selector7/2 -> PosMeas/2(GcHDP_IsoNegVolt_V)  "<GcHDP_IsoNegVolt_V>"
  Bus Selector7/3 -> PosMeas/3(GcHDP_PackVolt_V)  "<GcHDP_PackVolt_V>"
  Bus Selector8/2 -> NegMeas/2(GcHDP_IsoNegVolt_V)  "<GcHDP_IsoNegVolt_V>"
  Bus Selector8/1 -> NegMeas/1(LbISO_IsoForbid_flg)  "<LbISO_IsoForbid_flg>"
  Bus Selector8/3 -> NegMeas/3(GcHDP_PackVolt_V)  "<GcHDP_PackVolt_V>"
  ISO_GbISO_PosMosCmd_flg/1 -> GbISO_PosMosCmd_flg/1  "GbISO_PosMosCmd_flg"
  ISO_GbISO_NegMosCmd_flg/1 -> GbISO_NegMosCmd_flg/1  "GbISO_NegMosCmd_flg"
  ISOValueMeas/2(GbISO_ResCalFlt_flg) -> GbISO_ResCalFlt_flg/1
  Ground/1 -> ISO_GbISO_ResInitFlt_flg/1
  ISO_GbISO_ResInitFlt_flg/1 -> GbISO_ResInitFlt_flg/1  "GbISO_ResInitFlt_flg"
  GbNVM_ReadHVIsoValueVld_flg/1 -> Bus Creator/7
  Bus Selector/6 -> Initial/6(GbNVM_ReadHVIsoValueVld_flg)  "<GbNVM_ReadHVIsoValueVld_flg>"
  Bus Selector9/2 -> HVIsoMeasState/2(LbISO_IsoFastDetectEna_flg)  "<LbISO_IsoFastDetectEna_flg>"
  Bus Selector9/1 -> [LbISO_InitNegVoltCheck_flg], HVIsoMeasState/1(LbISO_InitNegVoltCheck_flg)  "<LbISO_InitNegVoltCheck_flg>"
  [LbISO_InitNegVoltCheck_flg] -> HVIsoValue/1(LbISO_InitNegVoltCheck_flg)
  Initial/1(LbISO_InitNegVoltCheck_flg) -> Bus Creator1/1
  Initial/2(LbISO_IsoFastDetectEna_flg) -> Bus Creator1/2
  Bus Creator1/1 -> Bus Selector9/1, Bus Selector10/1
  Bus Selector10/1 -> LbISO_InitNegVoltCheck_flg/1  "<LbISO_InitNegVoltCheck_flg>"
  Bus Selector10/2 -> LbISO_IsoFastDetectEna_flg/1  "<LbISO_IsoFastDetectEna_flg>"
  GcISP_ShutDownHVIsoValue_kohm/1 -> Bus Creator/8
  Bus Selector/7 -> Initial/7(GcISP_ShutDownHVIsoValue_kohm)  "<GcISP_ShutDownHVIsoValue_kohm>"
  Bus Selector11/1 -> HVIsoValue/2(GcISP_ShutDownHVIsoValue_kohm)  "<GcISP_ShutDownHVIsoValue_kohm>"
  Bus Selector11/2 -> HVIsoValue/3(GbNVM_ReadHVIsoValueVld_flg)  "<GbNVM_ReadHVIsoValueVld_flg>"

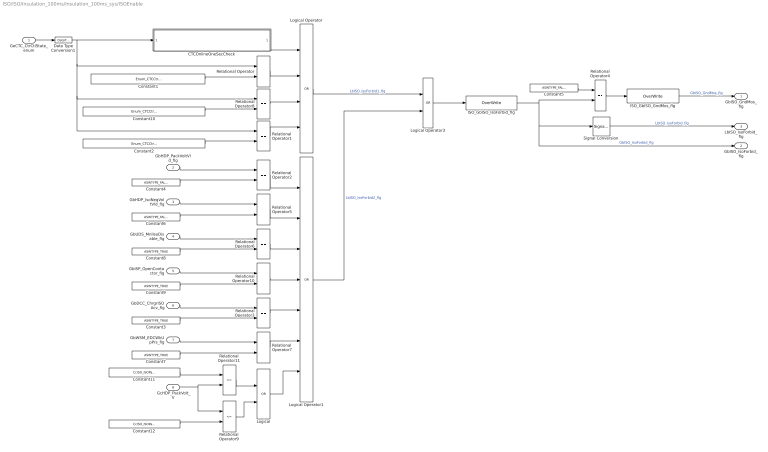
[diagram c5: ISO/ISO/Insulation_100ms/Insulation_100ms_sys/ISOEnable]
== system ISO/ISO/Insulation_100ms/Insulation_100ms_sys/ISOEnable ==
  GeCTC_CtrCtlState_enum : Inport
  GbHDP_PackVoltVld_flg : Inport  Port=2
  GbHDP_IsoNegVoltVld_flg : Inport  Port=3
  GbUDS_MnlIsoDisable_flg : Inport  Port=4
  GbISP_OpenContactor_flg : Inport  Port=5
  GbDCC_ChrgrISOAcv_flg : Inport  Port=6
  GbWSM_EDCWkUpPrs_flg : Inport  Port=7
  " GcHDP_PackVolt_V" : Inport  Port=8
  CTCOnlineOneSecCheck : Subsystem
  Constant1 : Constant  Value=Enum_CTCCtrCtlState.Enum_CTCCtrCtlState_Connect
  Constant10 : Constant  Value=Enum_CTCCtrCtlState.Enum_CTCCtrCtlState_PreShutdown
  Constant11 : Constant  Value=CcISO_ISOPackVoltMax_V
  Constant12 : Constant  Value=CcISO_ISOPackVoltMin_V
  Constant2 : Constant  Value=Enum_CTCCtrCtlState.Enum_CTCCtrCtlState_Shutdown
  Constant{3,7..9} (4 alike) : Constant  Value=ASWTYPE_TRUE
  Constant4 : Constant  Value=ASWTYPE_FALSE
  Constant5 : Constant  Value=ASWTYPE_FALSE
  Constant6 : Constant  Value=ASWTYPE_FALSE
  Data Type Conversion1 : DataTypeConversion
  ISO_GbISO_GndMos_flg : AIWAYS_Powertrain_BMS_lib/Signals/OverWrite  OverWrite_Value=CbISO_GndMosOvr_flg  OverWrite_flag=CbISO_GndMosOvrSwt_flg
  ISO_GbISO_IsoForbid_flg : AIWAYS_Powertrain_BMS_lib/Signals/OverWrite  OverWrite_Value=CbISO_IsoForbidOvr_flg  OverWrite_flag=CbISO_IsoForbidOvrSwt_flg
  Logical : Logic  Operator=OR  OutDataTypeStr=boolean
  Logical Operator : Logic  Operator=OR  Inputs=4  AllPortsSameDT=off  OutDataTypeStr=boolean
  Logical Operator1 : Logic  Operator=OR  Inputs=7  AllPortsSameDT=off  OutDataTypeStr=boolean
  Logical Operator3 : Logic  Operator=OR  AllPortsSameDT=off  OutDataTypeStr=boolean
  Relational Operator{,1..8,10} (10 alike) : RelationalOperator  Operator===  OutDataTypeStr=boolean
  Relational Operator11 : RelationalOperator  Operator=<=  OutDataTypeStr=boolean
  Relational Operator9 : RelationalOperator  Operator=<=  OutDataTypeStr=boolean
  Signal Conversion : SignalConversion  ConversionOutput=Contiguous copy  OverrideOpt=off
  GbISO_GndMos_flg : Outport
  GbISO_IsoForbid_flg : Outport  Port=2
  LbISO_IsoForbid_flg : Outport  Port=3
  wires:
  Constant1/1 -> Relational Operator/2
  Constant2/1 -> Relational Operator1/2
  GbHDP_PackVoltVld_flg/1 -> Relational Operator2/1
  Constant4/1 -> Relational Operator2/2
  GbHDP_IsoNegVoltVld_flg/1 -> Relational Operator5/1
  Constant6/1 -> Relational Operator5/2
  Logical Operator/1 -> Logical Operator3/1  "LbISO_IsoForbid1_flg"
  Logical Operator1/1 -> Logical Operator3/2  "LbISO_IsoForbid2_flg"
  GeCTC_CtrCtlState_enum/1 -> Data Type Conversion1/1
  GbUDS_MnlIsoDisable_flg/1 -> Relational Operator6/1
  Constant8/1 -> Relational Operator6/2
  Data Type Conversion1/1 -> CTCOnlineOneSecCheck/1(GeCTC_CtrCtlState_enum), Relational Operator/1, Relational Operator8/1, Relational Operator1/1
  Logical Operator3/1 -> ISO_GbISO_IsoForbid_flg/1
  Constant9/1 -> Relational Operator10/2
  GbISP_OpenContactor_flg/1 -> Relational Operator10/1
  CTCOnlineOneSecCheck/1(LbISO_CTCOnlineTimeReach_flg) -> Logical Operator/1
  Relational Operator/1 -> Logical Operator/2
  Relational Operator1/1 -> Logical Operator/4
  Constant3/1 -> Relational Operator3/2
  GbDCC_ChrgrISOAcv_flg/1 -> Relational Operator3/1
  Relational Operator2/1 -> Logical Operator1/1
  Relational Operator5/1 -> Logical Operator1/2
  Relational Operator6/1 -> Logical Operator1/3
  Relational Operator10/1 -> Logical Operator1/4
  Relational Operator3/1 -> Logical Operator1/5
  Constant5/1 -> Relational Operator4/1
  Relational Operator4/1 -> ISO_GbISO_GndMos_flg/1
  ISO_GbISO_GndMos_flg/1 -> GbISO_GndMos_flg/1  "GbISO_GndMos_flg"
  Constant7/1 -> Relational Operator7/2
  GbWSM_EDCWkUpPrs_flg/1 -> Relational Operator7/1
  Relational Operator7/1 -> Logical Operator1/6
  ISO_GbISO_IsoForbid_flg/1 -> Signal Conversion/1, GbISO_IsoForbid_flg/1, Relational Operator4/2  "GbISO_IsoForbid_flg"
  Constant10/1 -> Relational Operator8/2
  Relational Operator8/1 -> Logical Operator/3
  Signal Conversion/1 -> LbISO_IsoForbid_flg/1  "LbISO_IsoForbid_flg"
  Constant11/1 -> Relational Operator11/1
  " GcHDP_PackVolt_V"/1 -> Relational Operator9/1, Relational Operator11/2
  Constant12/1 -> Relational Operator9/2
  Relational Operator11/1 -> Logical/1
  Relational Operator9/1 -> Logical/2
  Logical/1 -> Logical Operator1/7

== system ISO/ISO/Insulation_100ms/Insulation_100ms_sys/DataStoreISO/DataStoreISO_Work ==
  GcISO_HVIsoValue_kohm : Inport
  Enable : EnablePort  StatesWhenEnabling=reset
  Data Store Write : AIWAYS_Powertrain_BMS_lib/Signals/Data Store Write  DSW=EcNVM_HVIsoValue_kohm
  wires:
  GcISO_HVIsoValue_kohm/1 -> Data Store Write/1

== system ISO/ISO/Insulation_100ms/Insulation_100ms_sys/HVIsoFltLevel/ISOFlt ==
  GcISO_HVIsoValue_kohm : Inport
  GeLDP_CC2St_enum : Inport  Port=2
  GeCTC_CtrCtlState_enum : Inport  Port=3
  LcISO_IsoSecondLevelResThrld_kohm : Inport  Port=4
  LcISO_IsoFirstLevelResThrld_kohm : Inport  Port=5
  LcISO_IsoNormalLevelResThrld_kohm : Inport  Port=6
  Bus Creator : BusCreator  Inputs=6
  Bus Creator2 : BusCreator  Inputs=6
  Bus Selector : BusSelector  OutputSignals=GcISO_HVIsoValue_kohm,GeLDP_CC2St_enum,GeCTC_CtrCtlState_enum,LcISO_IsoSecondLevelResThrld_kohm,LcISO_IsoFirstLevelResThrld_kohm,LcISO_IsoNormalLevelResThrld_kohm
  Bus Selector1 : BusSelector  OutputSignals=GcISO_HVIsoValue_kohm,GeCTC_CtrCtlState_enum,LcISO_IsoSecondLevelResThrld_kohm,LcISO_IsoFirstLevelResThrld_kohm,LcISO_IsoNormalLevelResThrld_kohm
  Bus Selector2 : BusSelector  OutputSignals=GcISO_HVIsoValue_kohm,GeLDP_CC2St_enum,LcISO_IsoSecondLevelResThrld_kohm,LcISO_IsoFirstLevelResThrld_kohm,LcISO_IsoNormalLevelResThrld_kohm,GeCTC_CtrCtlState_enum
  Bus Selector3 : BusSelector  OutputSignals=GbISO_IsoResFltLevel2_flg,GbISO_IsoResFltLevel1_flg,GbISO_IsoHVoffResFltLevel2_flg,GbISO_IsoHVoffResFltLevel1_flg,GbISO_IsoDCResFltLevel2_flg,GbISO_IsoDCResFltLevel1_flg
  Bus Selector4 : BusSelector  OutputSignals=GbISO_IsoResFltLevel2_flg,GbISO_IsoResFltLevel1_flg,GbISO_IsoHVoffResFltLevel2_flg,GbISO_IsoHVoffResFltLevel1_flg,GbISO_IsoDCResFltLevel2_flg,GbISO_IsoDCResFltLevel1_flg
  ISODCFlt : Subsystem
  ISOFltLevel : Subsystem
  ISOHVoffFlt : Subsystem
  ISOHVonFlt : Subsystem
  GeISO_ResFltLvl_enum : Outport
  GbISO_IsoResFltLevel1_flg : Outport  Port=2
  GbISO_IsoResFltLevel2_flg : Outport  Port=3
  GbISO_IsoResFltLevel3_flg : Outport  Port=4
  GbISO_IsoDCResFltLevel1_flg : Outport  Port=5
  GbISO_IsoDCResFltLevel2_flg : Outport  Port=6
  GbISO_IsoHVoffResFltLevel2_flg : Outport  Port=7
  GbISO_IsoHVoffResFltLevel1_flg : Outport  Port=8
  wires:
  GcISO_HVIsoValue_kohm/1 -> Bus Creator/1
  GeLDP_CC2St_enum/1 -> Bus Creator/2
  GeCTC_CtrCtlState_enum/1 -> Bus Creator/3
  LcISO_IsoSecondLevelResThrld_kohm/1 -> Bus Creator/4
  LcISO_IsoFirstLevelResThrld_kohm/1 -> Bus Creator/5
  LcISO_IsoNormalLevelResThrld_kohm/1 -> Bus Creator/6
  ISOFltLevel/1(GeISO_ResFltLvl_enum) -> GeISO_ResFltLvl_enum/1
  Bus Selector/1 -> ISOHVonFlt/1(GcISO_HVIsoValue_kohm)  "<GcISO_HVIsoValue_kohm>"
  Bus Selector/2 -> ISOHVonFlt/2(GeLDP_CC2St_enum)  "<GeLDP_CC2St_enum>"
  Bus Selector/3 -> ISOHVonFlt/3(GeCTC_CtrCtlState_enum)  "<GeCTC_CtrCtlState_enum>"
  Bus Selector/4 -> ISOHVonFlt/4(LcISO_IsoSecondLevelResThrld_kohm)  "<LcISO_IsoSecondLevelResThrld_kohm>"
  Bus Selector/5 -> ISOHVonFlt/5(LcISO_IsoFirstLevelResThrld_kohm)  "<LcISO_IsoFirstLevelResThrld_kohm>"
  Bus Selector/6 -> ISOHVonFlt/6(LcISO_IsoNormalLevelResThrld_kohm)  "<LcISO_IsoNormalLevelResThrld_kohm>"
  Bus Selector1/1 -> ISOHVoffFlt/1(GcISO_HVIsoValue_kohm)  "<GcISO_HVIsoValue_kohm>"
  Bus Selector1/2 -> ISOHVoffFlt/2(GeCTC_CtrCtlState_enum)  "<GeCTC_CtrCtlState_enum>"
  Bus Selector1/3 -> ISOHVoffFlt/3(LcISO_IsoSecondLevelResThrld_kohm)  "<LcISO_IsoSecondLevelResThrld_kohm>"
  Bus Selector1/4 -> ISOHVoffFlt/4(LcISO_IsoFirstLevelResThrld_kohm)  "<LcISO_IsoFirstLevelResThrld_kohm>"
  Bus Selector1/5 -> ISOHVoffFlt/5(LcISO_IsoNormalLevelResThrld_kohm)  "<LcISO_IsoNormalLevelResThrld_kohm>"
  Bus Creator/1 -> Bus Selector2/1, Bus Selector1/1, Bus Selector/1
  Bus Selector2/1 -> ISODCFlt/1(GcISO_HVIsoValue_kohm)  "<GcISO_HVIsoValue_kohm>"
  Bus Selector2/3 -> ISODCFlt/3(LcISO_IsoSecondLevelResThrld_kohm)  "<LcISO_IsoSecondLevelResThrld_kohm>"
  Bus Selector2/4 -> ISODCFlt/4(LcISO_IsoFirstLevelResThrld_kohm)  "<LcISO_IsoFirstLevelResThrld_kohm>"
  Bus Selector2/5 -> ISODCFlt/5(LcISO_IsoNormalLevelResThrld_kohm)  "<LcISO_IsoNormalLevelResThrld_kohm>"
  Bus Selector2/2 -> ISODCFlt/2(GeLDP_CC2St_enum)  "<GeLDP_CC2St_enum>"
  ISOHVonFlt/1(GbISO_IsoResFltLevel3_flg) -> GbISO_IsoResFltLevel3_flg/1
  ISOHVonFlt/2(GbISO_IsoResFltLevel2_flg) -> Bus Creator2/1
  ISOHVonFlt/3(GbISO_IsoResFltLevel1_flg) -> Bus Creator2/2
  ISOHVoffFlt/1(GbISO_IsoHVoffResFltLevel2_flg) -> Bus Creator2/3
  ISOHVoffFlt/2(GbISO_IsoHVoffResFltLevel1_flg) -> Bus Creator2/4
  ISODCFlt/1(GbISO_IsoDCResFltLevel2_flg) -> Bus Creator2/5
  ISODCFlt/2(GbISO_IsoDCResFltLevel1_flg) -> Bus Creator2/6
  Bus Creator2/1 -> Bus Selector4/1, Bus Selector3/1
  Bus Selector3/1 -> ISOFltLevel/1(GbISO_IsoResFltLevel2_flg)  "<GbISO_IsoResFltLevel2_flg>"
  Bus Selector3/2 -> ISOFltLevel/2(GbISO_IsoResFltLevel1_flg)  "<GbISO_IsoResFltLevel1_flg>"
  Bus Selector3/3 -> ISOFltLevel/3(GbISO_IsoHVoffResFltLevel2_flg)  "<GbISO_IsoHVoffResFltLevel2_flg>"
  Bus Selector3/4 -> ISOFltLevel/4(GbISO_IsoHVoffResFltLevel1_flg)  "<GbISO_IsoHVoffResFltLevel1_flg>"
  Bus Selector3/5 -> ISOFltLevel/5(GbISO_IsoDCResFltLevel2_flg)  "<GbISO_IsoDCResFltLevel2_flg>"
  Bus Selector3/6 -> ISOFltLevel/6(GbISO_IsoDCResFltLevel1_flg)  "<GbISO_IsoDCResFltLevel1_flg>"
  Bus Selector4/1 -> GbISO_IsoResFltLevel2_flg/1  "<GbISO_IsoResFltLevel2_flg>"
  Bus Selector4/2 -> GbISO_IsoResFltLevel1_flg/1  "<GbISO_IsoResFltLevel1_flg>"
  Bus Selector4/3 -> GbISO_IsoHVoffResFltLevel2_flg/1  "<GbISO_IsoHVoffResFltLevel2_flg>"
  Bus Selector4/4 -> GbISO_IsoHVoffResFltLevel1_flg/1  "<GbISO_IsoHVoffResFltLevel1_flg>"
  Bus Selector4/5 -> GbISO_IsoDCResFltLevel2_flg/1  "<GbISO_IsoDCResFltLevel2_flg>"
  Bus Selector4/6 -> GbISO_IsoDCResFltLevel1_flg/1  "<GbISO_IsoDCResFltLevel1_flg>"
  Bus Selector2/6 -> ISODCFlt/6(GeCTC_CtrCtlState_enum)  "<GeCTC_CtrCtlState_enum>"

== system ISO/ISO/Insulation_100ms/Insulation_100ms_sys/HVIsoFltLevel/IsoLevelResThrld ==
  GeCTC_CtrCtlState_enum : Inport
  GeCTC_CtrCtlConnMode_enum : Inport  Port=2
  Constant10 : Constant  Value=Enum_CTCCtrCtlConnMode.Enum_CTCCtrCtlConnMode_EDCChrg
  Constant19 : Constant  Value=CcISO_FirLvlResChrg_kohm
  Constant2 : Constant  Value=CcISO_SedLvlResChrg_kohm
  Constant3 : Constant  Value=CcISO_FirLvlResNotChrg_kohm
  Constant4 : Constant  Value=CcISO_SedLvlResNotChrg_kohm
  Constant5 : Constant  Value=CcISO_NorLvlResNotChrg_kohm
  Constant6 : Constant  Value=Enum_CTCCtrCtlConnMode.Enum_CTCCtrCtlConnMode_DCChrg
  Constant7 : Constant  Value=CcISO_NorLvlResChrg_kohm
  Constant8 : Constant  Value=Enum_CTCCtrCtlState.Enum_CTCCtrCtlState_Online
  Constant9 : Constant  Value=Enum_CTCCtrCtlConnMode.Enum_CTCCtrCtlConnMode_ACChrg
  Data Type Conversion1 : DataTypeConversion
  Data Type Conversion2 : DataTypeConversion
  Demux : Demux  Outputs=3
  Logical Operator2 : Logic  Operator=OR  Inputs=3  AllPortsSameDT=off  OutDataTypeStr=boolean
  Logical Operator4 : Logic  AllPortsSameDT=off  OutDataTypeStr=boolean
  Mux : Mux  Inputs=3
  Mux1 : Mux  Inputs=3
  Relational Operator{1..4} (4 alike) : RelationalOperator  Operator===  OutDataTypeStr=boolean
  Signal Conversion1 : SignalConversion  OverrideOpt=off
  Signal Conversion2 : SignalConversion  OverrideOpt=off
  Signal Conversion3 : SignalConversion  OverrideOpt=off
  Switch1 : Switch  Criteria=u2 ~= 0
  LcISO_IsoSecondLevelResThrld_kohm : Outport
  LcISO_IsoFirstLevelResThrld_kohm : Outport  Port=2
  LcISO_IsoNormalLevelResThrld_kohm : Outport  Port=3
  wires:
  Switch1/1 -> Demux/1
  Mux/1 -> Switch1/1
  Mux1/1 -> Switch1/3
  GeCTC_CtrCtlState_enum/1 -> Data Type Conversion1/1
  Constant2/1 -> Mux/1
  Constant19/1 -> Mux/2
  Constant7/1 -> Mux/3
  Signal Conversion1/1 -> LcISO_IsoSecondLevelResThrld_kohm/1  "LcISO_IsoSecondLevelResThrld_kohm"
  Signal Conversion2/1 -> LcISO_IsoFirstLevelResThrld_kohm/1  "LcISO_IsoFirstLevelResThrld_kohm"
  Signal Conversion3/1 -> LcISO_IsoNormalLevelResThrld_kohm/1  "LcISO_IsoNormalLevelResThrld_kohm"
  GeCTC_CtrCtlConnMode_enum/1 -> Data Type Conversion2/1
  Constant6/1 -> Relational Operator2/2
  Constant8/1 -> Relational Operator1/2
  Data Type Conversion1/1 -> Relational Operator1/1
  Constant9/1 -> Relational Operator3/2
  Data Type Conversion2/1 -> Relational Operator2/1, Relational Operator3/1, Relational Operator4/1
  Constant10/1 -> Relational Operator4/2
  Relational Operator2/1 -> Logical Operator2/1
  Relational Operator3/1 -> Logical Operator2/2
  Relational Operator4/1 -> Logical Operator2/3
  Logical Operator2/1 -> Logical Operator4/2
  Relational Operator1/1 -> Logical Operator4/1
  Logical Operator4/1 -> Switch1/2
  Demux/1 -> Signal Conversion1/1
  Demux/2 -> Signal Conversion2/1
  Demux/3 -> Signal Conversion3/1
  Constant4/1 -> Mux1/1
  Constant3/1 -> Mux1/2
  Constant5/1 -> Mux1/3

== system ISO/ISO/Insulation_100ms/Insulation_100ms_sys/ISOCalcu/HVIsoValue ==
  LbISO_InitNegVoltCheck_flg : Inport
  GcISP_ShutDownHVIsoValue_kohm : Inport  Port=2
  GbNVM_ReadHVIsoValueVld_flg : Inport  Port=3
  LbISO_ValueStEntry_flg : Inport  Port=4
  LcISO_HVIsoValue_kohm : Inport  Port=5
  Comparison4 : RelationalOperator  Operator===  OutDataTypeStr=boolean
  Constant1 : Constant  Value=CcISO_IsoDefaultValue_kohm
  Constant2 : Constant  Value=ASWTYPE_FALSE
  Constant3 : Constant  Value=CcISO_ISOResNvmMin_kohm
  Constant4 : Constant  Value=ISO_CONST0_NUMB
  Constant5 : Constant  Value=CcISO_IsoFastDectectInsVal_kohm
  EdgeFalling : AIWAYS_Powertrain_BMS_lib/Logical Operators/EdgeFalling
  EdgeRising : AIWAYS_Powertrain_BMS_lib/Logical Operators/EdgeRising
  ISOValueFilter : Subsystem
  ISO_GcISO_HVIsoValue_kohm : AIWAYS_Powertrain_BMS_lib/Signals/OverWrite  OverWrite_Value=CcISO_HVIsoValueOvr_kohm  OverWrite_flag=CbISO_HVIsoValueOvrSwt_flg
  Logical1 : Logic  Operator=OR  OutDataTypeStr=boolean
  Logical2 : Logic  Operator=OR  OutDataTypeStr=boolean
  MinMax1 : MinMax  Function=max  Inputs=2  OutDataTypeStr=Inherit: Inherit via back propagation  RndMeth=Zero
  Switch{1..4} (4 alike) : Switch  Criteria=u2 ~= 0
  Unit Delay2 : UnitDelay  SampleTime=-1  StateName=StateName
  Unit Delay21 : UnitDelay  InitialCondition=ASWTYPE_TRUE  SampleTime=-1  StateName=StateName
  GcISO_HVIsoValue_kohm : Outport
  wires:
  Switch3/1 -> ISO_GcISO_HVIsoValue_kohm/1
  ISO_GcISO_HVIsoValue_kohm/1 -> Unit Delay2/1, GcISO_HVIsoValue_kohm/1  "GcISO_HVIsoValue_kohm"
  GbNVM_ReadHVIsoValueVld_flg/1 -> Switch1/2
  GcISP_ShutDownHVIsoValue_kohm/1 -> MinMax1/2
  Constant1/1 -> Switch1/3
  Unit Delay21/1 -> Logical1/1
  Switch1/1 -> Switch3/1  "LcISO_HVIsoNvmValue_kohm"
  Constant2/1 -> Unit Delay21/1
  LbISO_ValueStEntry_flg/1 -> EdgeFalling/1
  LcISO_HVIsoValue_kohm/1 -> Switch2/3
  EdgeFalling/1 -> Logical2/1
  MinMax1/1 -> Switch1/1
  Constant3/1 -> MinMax1/1
  Constant4/1 -> Comparison4/1
  Logical1/1 -> Switch3/2  "LbISO_HVIsoNvmCalcSw_flg"
  Comparison4/1 -> Switch4/2, Logical1/2
  ISOValueFilter/1(LcISO_HVIsoValueFilter_kohm) -> Comparison4/2, Switch4/3
  LbISO_InitNegVoltCheck_flg/1 -> EdgeRising/1
  EdgeRising/1 -> Logical2/2, Switch2/2
  Logical2/1 -> ISOValueFilter/Enable
  Constant5/1 -> Switch2/1
  Switch2/1 -> ISOValueFilter/1(LcISO_HVIsoValue_kohm)
  Unit Delay2/1 -> Switch4/1
  Switch4/1 -> Switch3/3
